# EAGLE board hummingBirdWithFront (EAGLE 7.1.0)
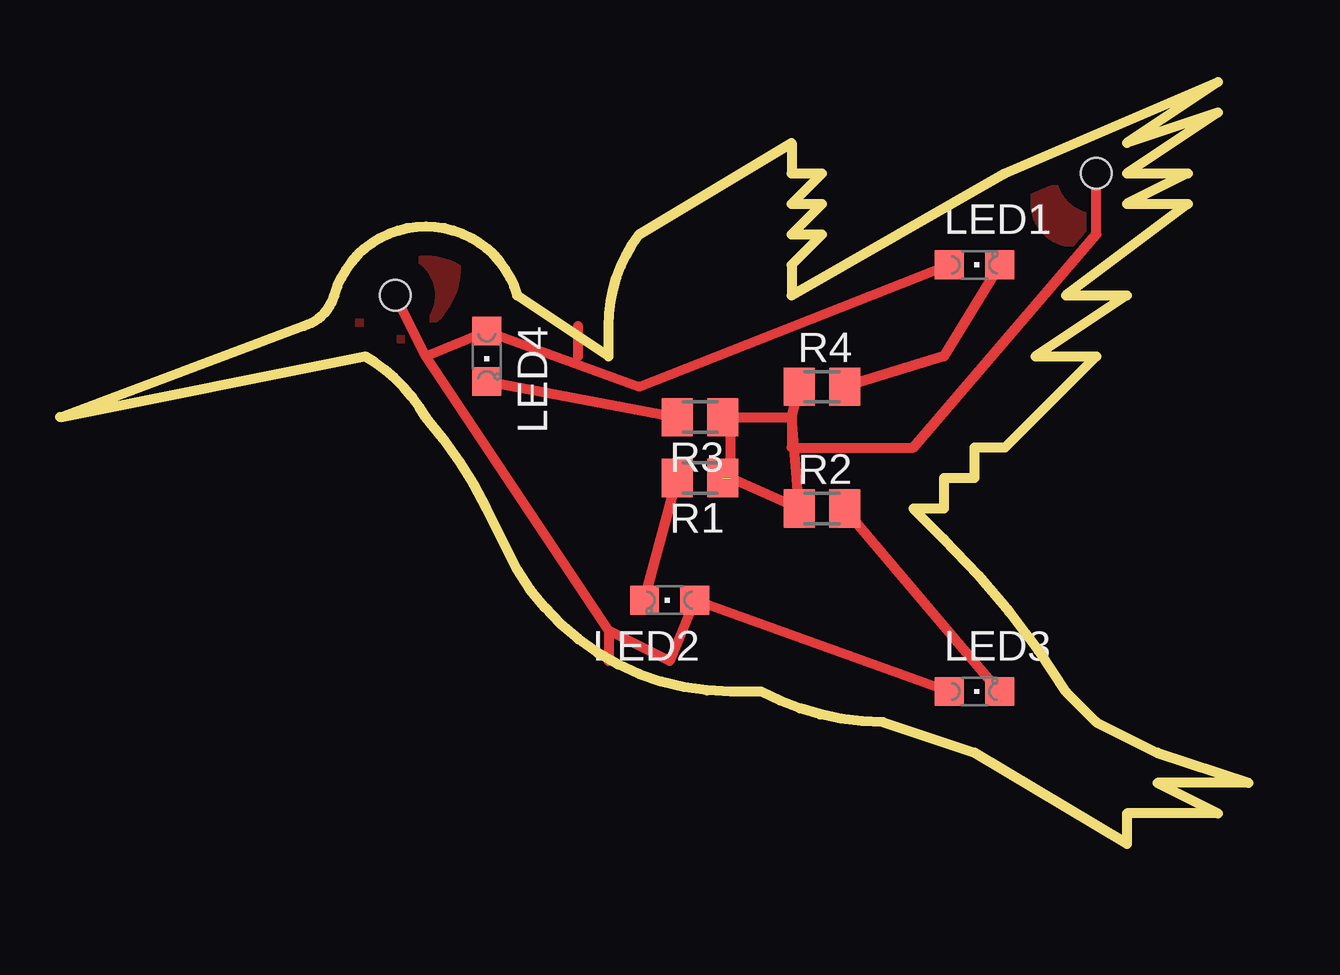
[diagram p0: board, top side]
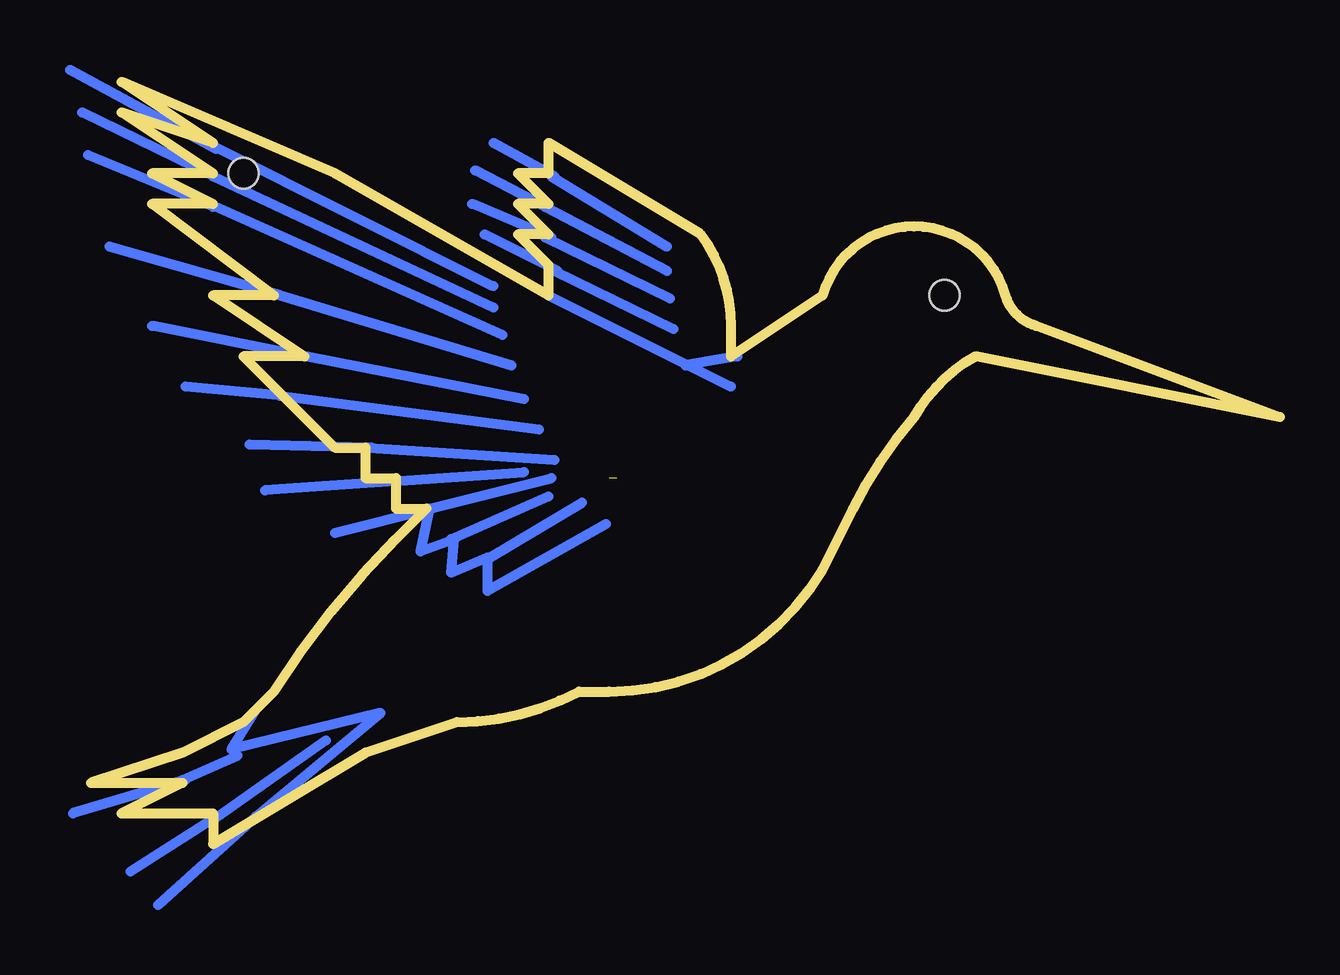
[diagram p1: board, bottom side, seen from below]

Size 49.53 x 31.75 mm. Coordinates in mm from the lower left corner, seen from the top.
Outline: 0,17.78 10.16,21.59 arc58 11.43,22.86 arc-148 19.05,22.86 22.86,20.32 22.86,21.59 arc-37 24.13,25.4 30.48,29.21 30.48,27.94 31.75,27.94 30.48,26.67 31.75,26.67 30.48,25.4 31.75,25.4 30.48,24.13 30.48,22.86 39.37,27.94 48.26,31.75 44.45,29.21 48.26,30.48 44.45,27.94 46.99,27.94 44.45,26.67 46.99,26.67 41.91,22.86 44.45,22.86 40.64,20.32 43.18,20.32 39.37,16.51 38.1,16.51 38.1,15.24 36.83,15.24 36.83,13.97 35.56,13.97 36.83,12.7 arc-13 41.91,6.35 43.18,5.08 45.72,3.81 49.53,2.54 45.72,2.54 48.26,1.27 44.45,1.27 44.45,0 38.1,3.81 34.29,5.08 arc-28 29.21,6.35 27.94,6.35 arc-59 19.05,11.43 17.78,13.97 arc14 15.24,17.78 arc31 12.7,20.32 0,17.78
Copper layers (1*16): Top 0.035mm / dielectric 1.5mm / Bottom 0.035mm
Design rules "default": minimum track width 10mil, minimum drill 24mil, track to track 8mil, track to pad 8mil, pad to pad 8mil, via to via 8mil, smd to smd 8mil, copper to edge 40mil, drill to drill 8mil, minimum pad ring 10mil, minimum via ring 8mil, stop-mask expansion 4mil, vias tented up to drill 0mil, thermal gap 10mil
Holes 1.27 mm at 13.97,22.86 43.18,27.94

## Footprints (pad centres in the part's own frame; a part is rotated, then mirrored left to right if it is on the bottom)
CHIPLED_0805 = smd 1.2 x 1.2: A 0,-1.05; C 0,1.05
M0805 = smd 1.3 x 1.6: 1 -0.95,0; 2 0.95,0

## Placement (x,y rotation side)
LED1  [CHIPLED_0805]  38.1,24.13 270 top
LED2  [CHIPLED_0805]  25.4,10.16 90 top
LED3  [CHIPLED_0805]  38.1,6.35 270 top
LED4  [CHIPLED_0805]  17.78,20.32 180 top
R1  [M0805]  26.67,15.24 180 top
R2  [M0805]  31.75,13.97 0 top
R3  [M0805]  26.67,17.78 180 top
R4  [M0805]  31.75,19.05 0 top

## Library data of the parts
LED1-LED4 = led
R1-R4 = resistor

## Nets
N$1: LED1.A LED2.A LED3.A LED4.A
N$2: LED2.C R1.2
N$3: LED3.C R2.2
N$4: LED4.C R3.2
N$5: LED1.C R4.2
N$6: R1.1 R2.1 R3.1 R4.1

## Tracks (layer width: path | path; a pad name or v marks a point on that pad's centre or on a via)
N$1
  Top 0.406: LED1.A 24.13,19.05 LED4.A 15.24,20.32 | LED3.A LED2.A 25.4,7.62 22.86,8.89 | 22.86,8.89 15.24,20.32 | 15.24,20.32 13.97,22.86 | 22.86,8.89 22.86,7.62
N$2
  Top 0.406: LED2.C R1.2
N$3
  Top 0.406: LED3.C R2.2
N$4
  Top 0.406: LED4.C R3.2
N$5
  Top 0.406: LED1.C 36.83,20.32 R4.2
N$6  (1 unrouted)
  Top 0.406: R3.1 27.94,17.78 | 27.94,17.78 30.48,17.78 | 30.48,17.78 R4.1 | 30.48,17.78 R2.1 27.94,15.24 27.94,17.78 | 30.48,17.78 30.48,16.51 35.56,16.51 43.18,25.4 43.18,27.94
N$7
  Top 0.406: 21.59,20.32 21.59,21.59
N$8
  pour Top: 13.97,25.4 15.24,25.4 arc-90 16.51,24.13 arc-53 15.24,21.59 arc-21 12.7,20.32 arc-159 11.43,22.86 arc16
N$9
  pour Top: 40.64,27.94 40.64,26.67 arc127 43.18,25.4 arc-21 45.72,26.67 arc184 44.45,30.48 arc26
N$10
  Bottom 0.406: 30.48,22.86 22.86,19.05
N$11
  Bottom 0.406: 22.61,20.32 24.77,19.94
N$12
  Bottom 0.406: 42.67,5.59 43.69,3.94 37.47,5.46 42.67,1.14 46.74,-2.54
N$13
  Bottom 0.406: 44.45,1.02 39.75,4.32
N$14
  Bottom 0.406: 45.72,2.67 43.43,3.68
N$15
  Bottom 0.406: 30.35,27.81 25.53,24.89
N$16
  Bottom 0.406: 25.53,23.88 30.61,26.54 33.53,28.07
N$17
  Bottom 0.406: 30.61,25.27 25.4,22.73
N$18
  Bottom 0.406: 30.23,23.88 25.27,21.46
N$19
  Bottom 0.406: 44.45,29.08 32.77,23.24
N$20
  Bottom 0.406: 32.77,22.35 44.45,27.81 49.91,30.48
N$21
  Bottom 0.406: 44.58,26.67 32.38,21.21
N$22
  Bottom 0.406: 32,19.94 41.66,22.86 48.77,24.89
N$23
  Bottom 0.406: 40.51,20.32 31.5,18.54
N$24
  Bottom 0.406: 41.66,18.67 30.86,17.27
N$25
  Bottom 0.406: 37.97,16.51 30.23,16
N$26
  Bottom 0.406: 28.07,13.33 33.02,10.54 33.02,11.94 34.54,11.3 34.42,12.7 35.81,12.19 35.43,13.97 30.35,15.24
N$27
  Bottom 0.406: 32.89,11.94 29.08,14.22
N$28
  Bottom 0.406: 34.54,12.7 30.48,14.48
N$29
  Bottom 0.406: 36.96,15.11 31.5,15.49
N$30
  Bottom 0.406: 30.23,27.81 32.77,29.21
N$31
  Bottom 0.406: 30.35,25.27 33.66,26.67
N$32
  Bottom 0.406: 30.1,23.88 33.15,25.4
N$33
  Bottom 0.406: 44.32,28.96 50.42,32.26
N$34
  Bottom 0.406: 44.45,26.54 49.66,28.7
N$35
  Bottom 0.406: 40.64,20.32 46.99,21.59
N$36
  Bottom 0.406: 41.53,18.67 45.59,19.05
N$37
  Bottom 0.406: 37.85,16.51 42.93,16.64
N$38
  Bottom 0.406: 36.83,15.11 42.29,14.73
N$39
  Bottom 0.406: 35.31,13.97 39.37,12.95
N$40
  Bottom 0.406: 45.59,2.67 50.29,1.27
N$41
  Bottom 0.406: 44.32,1.14 47.88,-1.14
(copper drawn outside any net)
  shapes: Bottom circle x1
